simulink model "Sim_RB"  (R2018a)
settings: Solver=ode45  StartTime=0.0  StopTime=30  RelTol=1e-3  EnableMultiTasking=on
InitFcn:
  | init;
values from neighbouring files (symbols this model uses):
  d2r = pi/180    (= 0.0174532925199)    [init.m]    (also in LQR_Design.m)
  r2d = 1/d2r    (= 57.2957795131)    [init.m]    (also in LQR_Design.m)
undefined symbols (not defined in the file or in its folder): Ad, Bd, Cd, Dd, Kpr, Kq, TVC

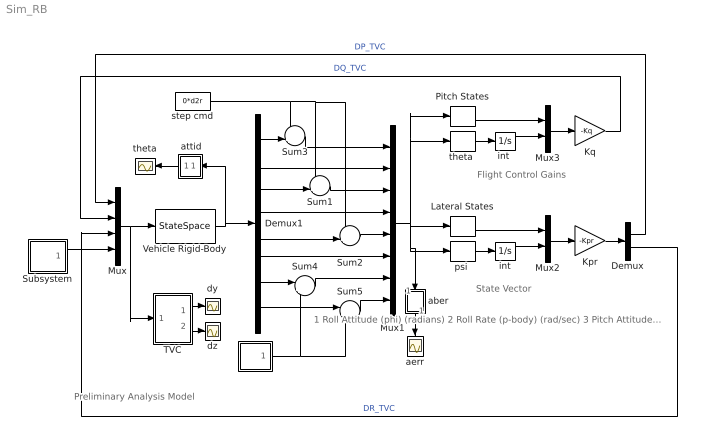
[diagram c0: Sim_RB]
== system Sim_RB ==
  note: 1 Roll Attitude (phi) (radians) 2 Roll Rate (p-body) (rad/sec) 3 Pitch Attitude (theta) (radians) 4 Pitch Rate (q-body) (rad/sec) 5 Yaw Attitude (psi) (radians) 6 Yaw Rate (r-body) (rad/sec) 7 Angle of attack, alfa, (radians) 8 Angle of sideslip, beta, (radian)
  note: Flight Control Gains
  note: State Vector
  note: Preliminary Analysis Model
  "  " : Subsystem
  " attid" : Subsystem
  Demux : Demux  Outputs=2
  Demux1 : Demux  Outputs=8
  Kpr : Gain  Gain=-Kpr  Multiplication=Matrix(K*u)
  Kq : Gain  Gain=-Kq  Multiplication=Matrix(K*u)
  Lateral States : Selector  InputPortWidth=8  IndexOptions=Index vector (dialog)  Indices="[1  2  5  6  8]"  OutputSizes=1
  Mux : Mux
  Mux1 : Mux  Inputs=8
  Mux2 : Mux  Inputs=[5, 1]
  Mux3 : Mux  Inputs=[3, 1]
  Pitch States : Selector  InputPortWidth=8  IndexOptions=Index vector (dialog)  Indices="[3  4  7]"  OutputSizes=1
  Subsystem : Subsystem
  Sum1 : Sum  Inputs=-+|
  Sum2 : Sum  Inputs=-+|
  Sum3 : Sum  Inputs=-+|
  Sum4 : Sum  Inputs=|++
  Sum5 : Sum  Inputs=|++
  TVC : Subsystem
  Vehicle Rigid-Body : StateSpace  A=Ad  B=Bd  C=Cd  D=Dd  InitialCondition=0
  aber : Subsystem
  aerr : Scope
  dy : Scope
  dz : Scope
  int : Integrator
  "int " : Integrator
  "psi " : Selector  InputPortWidth=8  IndexOptions=Index vector (dialog)  Indices=[5]  OutputSizes=1
  step cmd : Constant  Value=0*d2r
  theta : Scope
  "theta " : Selector  InputPortWidth=8  IndexOptions=Index vector (dialog)  Indices=[3]  OutputSizes=1
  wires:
  Mux/1 -> TVC/1(tvc), Vehicle Rigid-Body/1
  Vehicle Rigid-Body/1 -> " attid"/1(i), Demux1/1
  Demux1/6 -> Mux1/6
  Demux1/4 -> Mux1/4
  Demux1/2 -> Mux1/2
  Demux1/3 -> Sum1/2
  Sum1/1 -> Mux1/3
  Demux1/5 -> Sum2/2
  Sum2/1 -> Mux1/5
  Mux1/1 -> "theta "/1, Pitch States/1, "psi "/1, aber/1(i), Lateral States/1
  Demux/1 -> Mux/1  "DP_TVC"
  Kpr/1 -> Demux/1
  Kq/1 -> Mux/2  "DQ_TVC"
  Mux2/1 -> Kpr/1
  Lateral States/1 -> Mux2/1
  int/1 -> Mux2/2
  "psi "/1 -> int/1
  Demux1/1 -> Sum3/2
  Sum3/1 -> Mux1/1
  step cmd/1 -> Sum3/1, Sum2/1, Sum1/1
  TVC/1(dy) -> dy/1
  TVC/2(dz) -> dz/1
  Demux/2 -> Mux/3  "DR_TVC"
  " attid"/1(o) -> theta/1
  Demux1/7 -> Sum4/1
  Sum4/1 -> Mux1/7
  Sum5/1 -> Mux1/8
  Demux1/8 -> Sum5/1
  "  "/1(alpha) -> Sum5/2, Sum4/2
  aber/1(o) -> aerr/1
  "int "/1 -> Mux3/2
  "theta "/1 -> "int "/1
  Pitch States/1 -> Mux3/1
  Mux3/1 -> Kq/1
  Subsystem/1(Gust) -> Mux/4

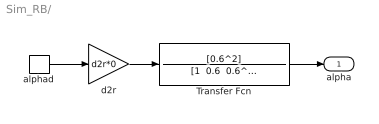
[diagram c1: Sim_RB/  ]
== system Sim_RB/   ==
  Transfer Fcn : TransferFcn  Numerator=[0.6^2]  Denominator="[1  0.6  0.6^2]"
  alphad : DiscretePulseGenerator  PulseType=Time based  Amplitude=5  Period=200  PulseWidth=5  PhaseDelay=2
  d2r : Gain  Gain=d2r*0
  alpha : Outport
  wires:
  alphad/1 -> d2r/1
  Transfer Fcn/1 -> alpha/1
  d2r/1 -> Transfer Fcn/1

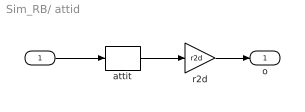
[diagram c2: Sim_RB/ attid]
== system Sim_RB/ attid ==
  i : Inport
  attit : Selector  InputPortWidth=8  IndexOptions=Index vector (dialog)  Indices="[1  3   5]"  OutputSizes=1
  r2d : Gain  Gain=r2d
  o : Outport
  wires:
  attit/1 -> r2d/1
  r2d/1 -> o/1
  i/1 -> attit/1

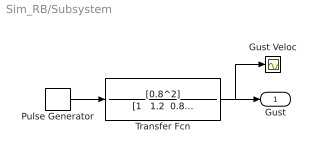
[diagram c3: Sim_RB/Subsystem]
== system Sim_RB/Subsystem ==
  Gust Veloc : Scope
  Pulse Generator : DiscretePulseGenerator  PulseType=Time based  Amplitude=30  Period=200  PulseWidth=10
  Transfer Fcn : TransferFcn  Numerator=[0.8^2]  Denominator="[1   1.2  0.8^2]"
  Gust : Outport
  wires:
  Transfer Fcn/1 -> Gust Veloc/1, Gust/1
  Pulse Generator/1 -> Transfer Fcn/1

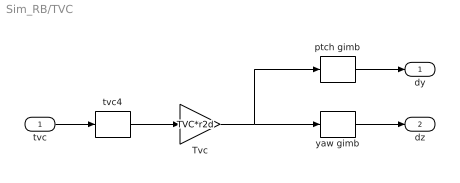
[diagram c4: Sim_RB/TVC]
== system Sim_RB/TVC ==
  tvc : Inport
  Tvc : Gain  Gain=TVC*r2d  Multiplication=Matrix(K*u)
  ptch gimb : Selector  InputPortWidth=16  IndexOptions=Index vector (dialog)  Indices=[1:8]  OutputSizes=1
  tvc4 : Selector  InputPortWidth=4  IndexOptions=Index vector (dialog)  Indices=[1:3]  OutputSizes=1
  yaw gimb : Selector  InputPortWidth=16  IndexOptions=Index vector (dialog)  Indices=[9:16]  OutputSizes=1
  dy : Outport
  dz : Outport  Port=2
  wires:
  Tvc/1 -> ptch gimb/1, yaw gimb/1
  tvc/1 -> tvc4/1
  ptch gimb/1 -> dy/1
  yaw gimb/1 -> dz/1
  tvc4/1 -> Tvc/1

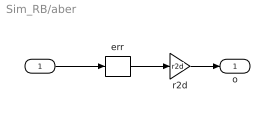
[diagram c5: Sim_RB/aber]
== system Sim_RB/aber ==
  i : Inport
  err : Selector  InputPortWidth=8  IndexOptions=Index vector (dialog)  Indices=[7:8]  OutputSizes=1
  r2d : Gain  Gain=r2d
  o : Outport
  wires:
  r2d/1 -> o/1
  err/1 -> r2d/1
  i/1 -> err/1
